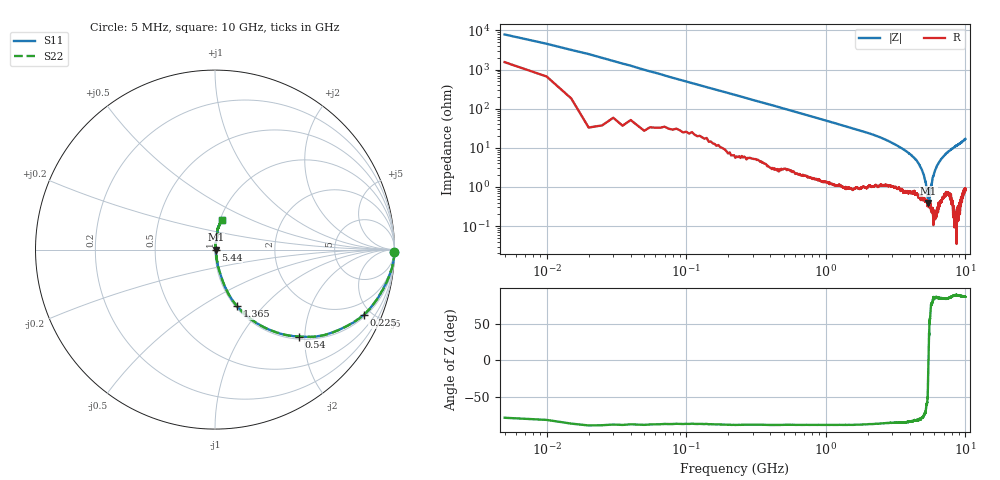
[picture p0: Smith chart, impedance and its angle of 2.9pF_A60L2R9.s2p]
! Amotech Co.,Ltd.
! http://www.amotech.co.kr/
! Part Number: A60L2R9
! These Parameters are Measured in Series Mode Connection
! Operation Temp=25[degC], DC Bias Voltage=0[V]
! Freq. Start=5[MHz] Stop=10[GHz], 2000[Steps]
! Date: Monday, July 14, 2020, 09:49:02
# GHZ S RI R 50.000000
!Freq.(Hz) S11(Real) S11(Imag) S21(Real) S21(Imag) S12(Real) S12(Imag) S22(Real) S22(Imag)
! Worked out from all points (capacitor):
!   2000 points, 5 MHz to 10 GHz, reference 50 ohm
!   read as one part in series: C = 3.22 pF near 55 MHz
!   lowest |Z| = 390 mohm at 5.415 GHz (marker M1)
!   series resonance near 5.44 GHz, so ESL is about 270 pH
!   S11 on the Smith chart (normalised r, x): 5 MHz: open; 225 MHz: 1.11, -4.47; 540 MHz: 1.06, -1.86; 1.365 GHz: 1.02, -0.73; 5.44 GHz: 1.01, -0.00; 10 GHz: 1.02, +0.34
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0.005  0.9974 -0.0123  0.00263 0.0123  0.00263 0.0123  0.9974 -0.0123
0.065  0.9782 -0.1264  0.0218 0.1264  0.0218 0.1264  0.9782 -0.1264
0.09  0.9598 -0.1726  0.0402 0.1726  0.0402 0.1726  0.9598 -0.1726
0.145  0.9126 -0.2623  0.0874 0.2623  0.0874 0.2623  0.9126 -0.2623
0.225  0.8275 -0.3656  0.1725 0.3656  0.1725 0.3656  0.8275 -0.3656
0.54  0.4655 -0.4842  0.5345 0.4842  0.5345 0.4842  0.4655 -0.4842
0.89  0.2464 -0.4173  0.7536 0.4173  0.7536 0.4173  0.2464 -0.4173
1.365  0.1225 -0.3155  0.8775 0.3155  0.8775 0.3155  0.1225 -0.3155
1.675  0.0862 -0.2646  0.9138 0.2646  0.9138 0.2646  0.0862 -0.2646
3.34  0.0206 -0.1035  0.9794 0.1035  0.9794 0.1035  0.0206 -0.1035
4.455  0.00915 -0.0476  0.9908 0.0476  0.9908 0.0476  0.00915 -0.0476
5.005  0.00529 -0.0206  0.9947 0.0206  0.9947 0.0206  0.00529 -0.0206
5.21  0.00461 -0.011  0.9954 0.011  0.9954 0.011  0.00461 -0.011
5.415  0.00369 -0.00122  0.9963 0.00122  0.9963 0.00122  0.00369 -0.00122
5.44  0.00396 -9.82e-06  0.996 9.82e-06  0.996 9.82e-06  0.00396 -9.82e-06
5.51  0.00337 0.00285  0.9966 -0.00285  0.9966 -0.00285  0.00337 0.00285
5.645  0.00351 0.00911  0.9965 -0.00911  0.9965 -0.00911  0.00351 0.00911
5.86  0.00258 0.0179  0.9974 -0.0179  0.9974 -0.0179  0.00258 0.0179
6.265  0.00406 0.0348  0.9959 -0.0348  0.9959 -0.0348  0.00406 0.0348
6.67  0.0069 0.0494  0.9931 -0.0494  0.9931 -0.0494  0.0069 0.0494
8.335  0.0121 0.1037  0.9879 -0.1037  0.9879 -0.1037  0.0121 0.1037
10  0.0365 0.1625  0.9635 -0.1625  0.9635 -0.1625  0.0365 0.1625
